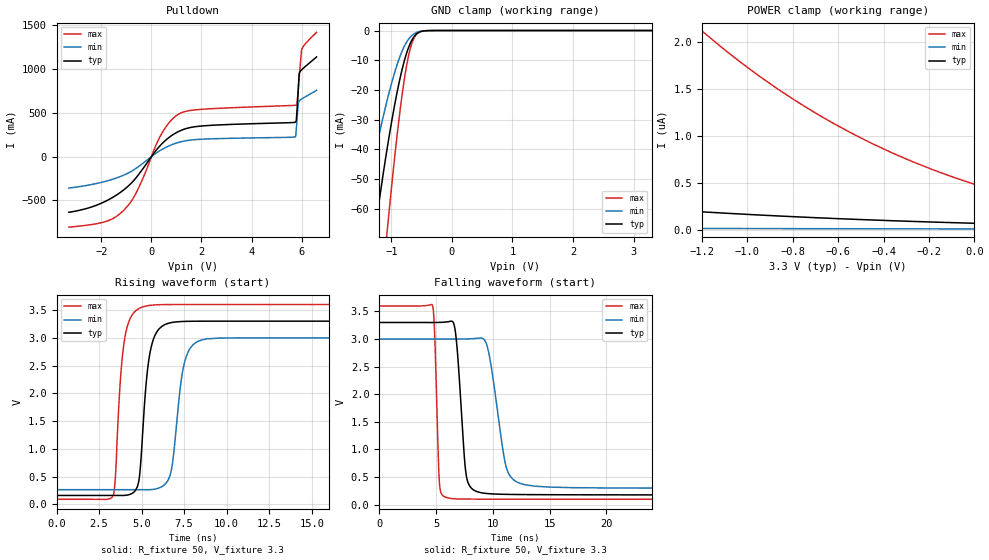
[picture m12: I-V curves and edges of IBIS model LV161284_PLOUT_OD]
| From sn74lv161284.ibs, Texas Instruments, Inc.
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[Model]   LV161284_PLOUT_OD
Model_type  Open_drain
Enable   Active-Low
Vref =   3.3
Rref =   500
Cref =   50p
Vmeas =   1.4
| variable   typ   min   max
C_comp   6.22pF   5.00pF   7.25pF
| C_pulldown   9.97pF   6.01pF   13.91pF
| C_tri-state   6.22pF   5.00pF   7.25pF
[Temperature Range]   40   100   -40
| Ambient temperature   25   85   -40
[Voltage range]   3.3   3   3.6
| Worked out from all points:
|   slope of the pulldown table from 0 to 0.495 V, typ, clamps not added: 2.94 ohm
|   GND clamp passes 1 mA (typ) near -0.58 V on its own axis
|   rising waveform, R_fixture 50, V_fixture 3.3: 20-80 % time 504ps typ, 602ps min, 451ps max; typ from 0.161 V to 3.3 V
|   falling waveform, R_fixture 50, V_fixture 3.3: 20-80 % time 603ps typ, 1.12ns min, 300ps max; typ from 3.3 V to 0.171 V
[GND Clamp]
| LV161284_PLOUT_OD
|   Voltage   I(typ)   I(min)   I(max)
-3.3V     -487.8mA   -311.1mA   -672.5mA
-1.545V   -112mA     -69.95mA   -181mA
-1.505V   -105.1mA   -65.56mA   -170.8mA
-1.27V    -67.57mA   -41.43mA   -113mA
-1.065V   -39.19mA   -23.14mA   -66.84mA
-925mV    -22.88mA   -12.79mA   -38.95mA
-800mV    -11.32mA   -5.911mA   -18.44mA
-700mV    -4.919mA   -2.51mA    -7.105mA
-650mV    -2.828mA   -1.491mA   -3.693mA
-590mV    -1.25mA    -727.3uA   -1.405mA
-390mV    -34.43uA   -25.54uA   -18.53uA
3.3V      69.14nA    9.916nA    287.2nA
[POWER Clamp]
| LV161284_PLOUT_OD
|   Voltage   I(typ)   I(min)   I(max)
-3.3V     4.888uA    865.6nA    23.79uA
-3.16V    3.438uA    342.4nA    19.91uA
-3.005V   2.146uA    82.16nA    16.1uA
-2.885V   1.39uA     33.66nA    13.49uA
-2.78V    920.3nA    24.78nA    11.48uA
-2.675V   642.3nA    22.5nA     9.718uA
-2.56V    513.7nA    21.51nA    8.087uA
-1.18V    188.3nA    13.38nA    2.079uA
-945mV    156.9nA    12.44nA    1.634uA
-620mV    120.3nA    11.16nA    1.133uA
-360mV    96.18nA    10.15nA    817.4nA
-48.03fV  69.14nA    8.749nA    485.3nA
[Pulldown]
| LV161284_PLOUT_OD
|   Voltage   I(typ)   I(min)   I(max)
-3.3V     -636.8mA   -359.6mA   -806.4mA
-1.825V   -509mA     -281.8mA   -741.7mA
-1.08V    -373.7mA   -208.2mA   -604.8mA
-570mV    -225.9mA   -125mA     -390.6mA
415mV     145.6mA    81.03mA    266mA
1.115V    290.9mA    164.5mA    490.4mA
5.705V    390.1mA    223mA      585.4mA
5.765V    396.2mA    234.7mA    587.6mA
5.8V      457.2mA    356mA      592.9mA
5.905V    946.2mA    636.8mA    895.5mA
6.01V     993.9mA    659.3mA    1.226A
6.6V      1.139A     756.9mA    1.42A
[Ramp]
| LV161284_PLOUT_OD
| variable   typ   min   max
dV/dt_r   1.88/5.07E-10   1.64/6.04E-10   2.11/4.60E-10
dV/dt_f   1.89/6.12E-10   1.64/1.13E-09   2.12/3.10E-10
R_load = 50
[Rising Waveform]
| LV161284_PLOUT_OD
R_fixture =   50
C_fixture =   0
L_fixture =   0
V_fixture =   3.3
V_fixture_min = 3
V_fixture_max = 3.6
|   Time   V(typ)   V(min)   V(max)
0s        161.3mV    265mV      91.9mV
3.33ns    161.3mV    265mV      163.8mV
3.775ns   160.7mV    265mV      2.332V
4.03ns    162.4mV    265mV      3.029V
4.845ns   434mV      264.6mV    3.528V
5.375ns   2.491V     264.2mV    3.58V
6.64ns    3.268V     495mV      3.6V
7.535ns   3.296V     2.572V     3.601V
8.835ns   3.3V       2.981V     3.601V
70ns      3.3V       3V         3.6V
[Falling Waveform]
| LV161284_PLOUT_OD
R_fixture =   50
C_fixture =   0
L_fixture =   0
V_fixture =   3.3
V_fixture_min = 3
V_fixture_max = 3.6
|   Time   V(typ)   V(min)   V(max)
0s        3.3V       3V         3.6V
4.67ns    3.299V     3V         3.617V
5.305ns   3.301V     3V         375.1mV
6.01ns    3.312V     2.999V     120.1mV
6.73ns    3.09V      3V         103.1mV
7.69ns    494.4mV    3.002V     98.99mV
8.835ns   220.3mV    3.018V     97.75mV
11.21ns   184.2mV    657.1mV    96.67mV
12.84ns   180.3mV    358.4mV    96.29mV
70ns      171.1mV    287.6mV    94.22mV
